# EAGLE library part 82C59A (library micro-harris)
MICROCONTROLLER/MEMORY DEVICE
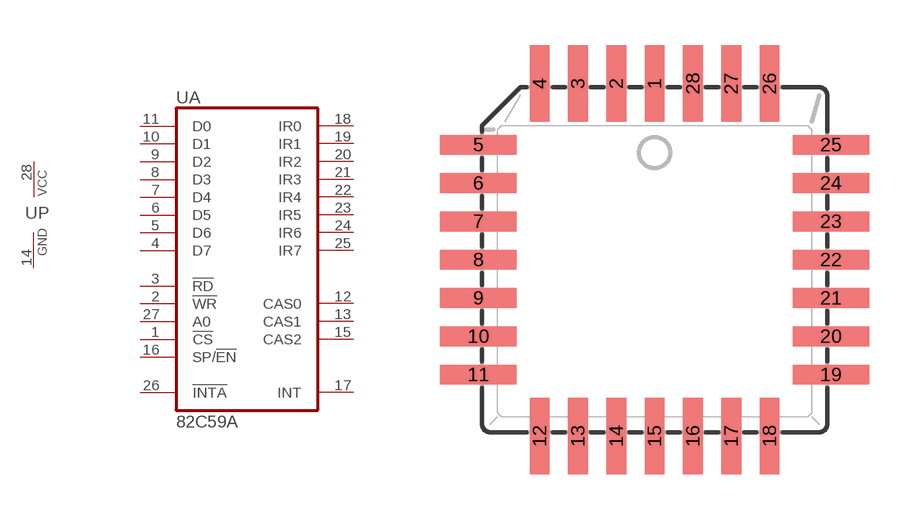
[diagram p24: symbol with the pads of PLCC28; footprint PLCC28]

Designator prefix U; gates A=82C59A P=PWRN

## 82C59A (MF: INTERSIL; MPN: IS82C59A; OC_FARNELL: unknown; OC_NEWARK: 05B7426)  [PLCC28]
1  A:!CS  in
2  A:!WR  in
3  A:!RD  in
4  A:D7
5  A:D6
6  A:D5
7  A:D4
8  A:D3
9  A:D2
10  A:D1
11  A:D0
12  A:CAS0
13  A:CAS1
14  P:GND  pwr
15  A:CAS2
16  A:SP/!EN
17  A:INT  out
18  A:IR0  in
19  A:IR1  in
20  A:IR2  in
21  A:IR3  in
22  A:IR4  in
23  A:IR5  in
24  A:IR6  in
25  A:IR7  in
26  A:!INTA  in
27  A:A0  in
28  P:VCC  pwr

## Footprint PLCC28 (pad centres in mm)
PLASTIC LEADED CHIP CARRIER square
smd 0.66 x 2.54: 1 0,5.842; 2 -1.27,5.842; 3 -2.54,5.842; 4 -3.81,5.842; 12 -3.81,-5.842; 13 -2.54,-5.842; 14 -1.27,-5.842; 15 0,-5.842; 16 1.27,-5.842; 17 2.54,-5.842; 18 3.81,-5.842; 26 3.81,5.842; 27 2.54,5.842; 28 1.27,5.842
smd 2.54 x 0.66: 5 -5.842,3.81; 6 -5.842,2.54; 7 -5.842,1.27; 8 -5.842,0; 9 -5.842,-1.27; 10 -5.842,-2.54; 11 -5.842,-3.81; 19 5.842,-3.81; 20 5.842,-2.54; 21 5.842,-1.27; 22 5.842,0; 23 5.842,1.27; 24 5.842,2.54; 25 5.842,3.81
